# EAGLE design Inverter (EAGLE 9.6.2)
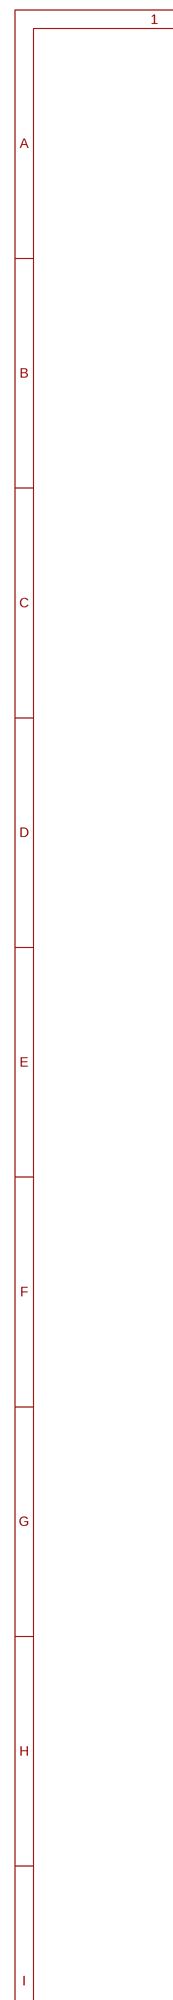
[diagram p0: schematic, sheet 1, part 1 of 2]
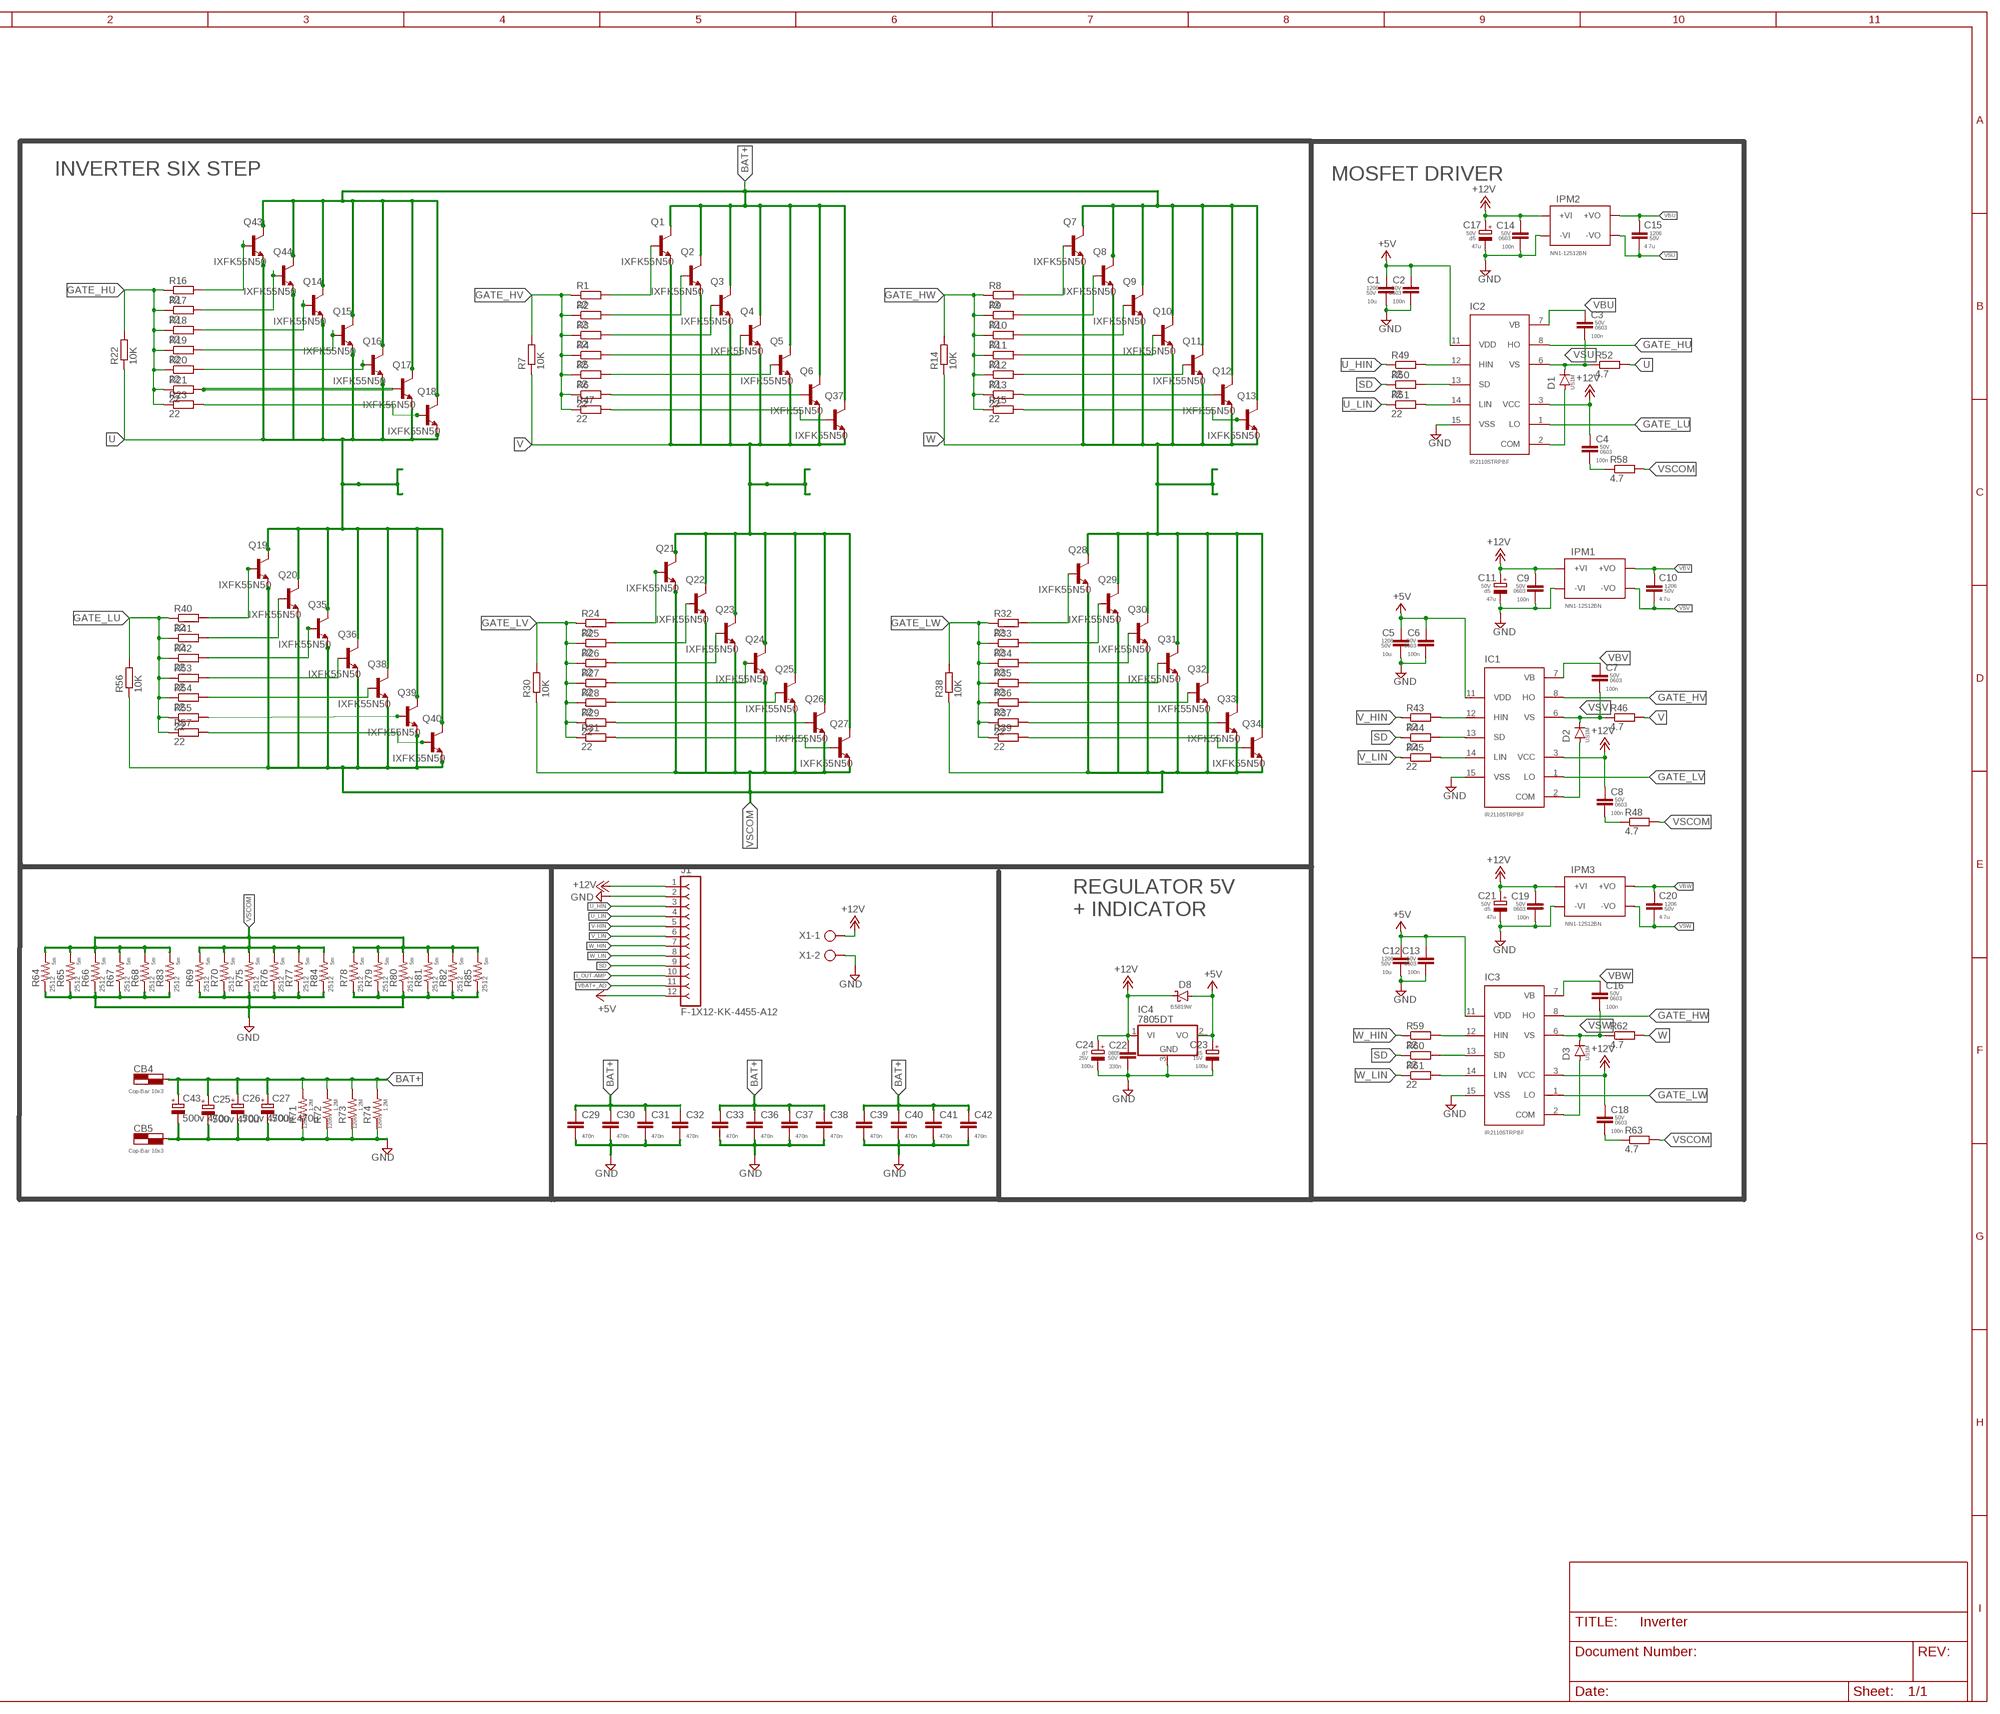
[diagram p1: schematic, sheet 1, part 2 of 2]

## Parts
C1  10u  C-EUC1206  [C1206]
C2  100n  C-EUC0603  [C0603]
C3  100n  C-EUC0603  [C0603]
C4  100n  C-EUC0603  [C0603]
C5  10u  C-EUC1206  [C1206]
C6  100n  C-EUC0603  [C0603]
C7  100n  C-EUC0603  [C0603]
C8  100n  C-EUC0603  [C0603]
C9  100n  C-EUC0603  [C0603]
C10  4.7u  C-EUC1206  [C1206]
C11  47u  CPOL-EUE2.5-5  [E2,5-5]
C12  10u  C-EUC1206  [C1206]
C13  100n  C-EUC0603  [C0603]
C14  100n  C-EUC0603  [C0603]
C15  4.7u  C-EUC1206  [C1206]
C16  100n  C-EUC0603  [C0603]
C17  47u  CPOL-EUE2.5-5  [E2,5-5]
C18  100n  C-EUC0603  [C0603]
C19  100n  C-EUC0603  [C0603]
C20  4.7u  C-EUC1206  [C1206]
C21  47u  CPOL-EUE2.5-5  [E2,5-5]
C22  330n  C-EUC0805  [C0805]
C23  100u  CPOL-EUE2.5-5  [E2,5-5]
C24  100u  CPOL-EUE2.5-7  [E2,5-7]
C25  500v 470u  CPOL-EUE10-35  [EB35D]
C26  500v 470u  CPOL-EUE10-35  [EB35D]
C27  500v 470u  CPOL-EUE10-35  [EB35D]
C29  470n  C-EU102-064X133  [C102-064X133]
C30  470n  C-EU102-064X133  [C102-064X133]
C31  470n  C-EU102-064X133  [C102-064X133]
C32  470n  C-EU102-064X133  [C102-064X133]
C33  470n  C-EU102-064X133  [C102-064X133]
C36  470n  C-EU102-064X133  [C102-064X133]
C37  470n  C-EU102-064X133  [C102-064X133]
C38  470n  C-EU102-064X133  [C102-064X133]
C39  470n  C-EU102-064X133  [C102-064X133]
C40  470n  C-EU102-064X133  [C102-064X133]
C41  470n  C-EU102-064X133  [C102-064X133]
C42  470n  C-EU102-064X133  [C102-064X133]
C43  500v 470u  CPOL-EUE10-35  [EB35D]
CB4  Cop-Bar 10x3  COOPPER_BAR15X2  [COP_BAR-15X2]
CB5  Cop-Bar 10x3  COOPPER_BAR15X2  [COP_BAR-15X2]
D1  US1M  GF1  [SMA-DO214AC]
D2  US1M  GF1  [SMA-DO214AC]
D3  US1M  GF1  [SMA-DO214AC]
D8  B5819W  SCHOTTKY-DIODESOD123  [DIODE_SOD123]
IC1  IR2110STRPBF  IR2110  [SO16W]
IC2  IR2110STRPBF  IR2110  [SO16W]
IC3  IR2110STRPBF  IR2110  [SO16W]
IC4  7805DT  [TO252]
IPM1  NN1-12S12BN  [NN1-12S12BN]
IPM2  NN1-12S12BN  [NN1-12S12BN]
IPM3  NN1-12S12BN  [NN1-12S12BN]
J1  F-1X12-KK-4455-A12  [KK-4455-A12]
Q1  IXFK55N50  2SC5200  [TO545P2020X520X2910-3]
Q2  IXFK55N50  2SC5200  [TO545P2020X520X2910-3]
Q3  IXFK55N50  2SC5200  [TO545P2020X520X2910-3]
Q4  IXFK55N50  2SC5200  [TO545P2020X520X2910-3]
Q5  IXFK55N50  2SC5200  [TO545P2020X520X2910-3]
Q6  IXFK55N50  2SC5200  [TO545P2020X520X2910-3]
Q7  IXFK55N50  2SC5200  [TO545P2020X520X2910-3]
Q8  IXFK55N50  2SC5200  [TO545P2020X520X2910-3]
Q9  IXFK55N50  2SC5200  [TO545P2020X520X2910-3]
Q10  IXFK55N50  2SC5200  [TO545P2020X520X2910-3]
Q11  IXFK55N50  2SC5200  [TO545P2020X520X2910-3]
Q12  IXFK55N50  2SC5200  [TO545P2020X520X2910-3]
Q13  IXFK55N50  2SC5200  [TO545P2020X520X2910-3]
Q14  IXFK55N50  2SC5200  [TO545P2020X520X2910-3]
Q15  IXFK55N50  2SC5200  [TO545P2020X520X2910-3]
Q16  IXFK55N50  2SC5200  [TO545P2020X520X2910-3]
Q17  IXFK55N50  2SC5200  [TO545P2020X520X2910-3]
Q18  IXFK55N50  2SC5200  [TO545P2020X520X2910-3]
Q19  IXFK55N50  2SC5200  [TO545P2020X520X2910-3]
Q20  IXFK55N50  2SC5200  [TO545P2020X520X2910-3]
Q21  IXFK55N50  2SC5200  [TO545P2020X520X2910-3]
Q22  IXFK55N50  2SC5200  [TO545P2020X520X2910-3]
Q23  IXFK55N50  2SC5200  [TO545P2020X520X2910-3]
Q24  IXFK55N50  2SC5200  [TO545P2020X520X2910-3]
Q25  IXFK55N50  2SC5200  [TO545P2020X520X2910-3]
Q26  IXFK55N50  2SC5200  [TO545P2020X520X2910-3]
Q27  IXFK55N50  2SC5200  [TO545P2020X520X2910-3]
Q28  IXFK55N50  2SC5200  [TO545P2020X520X2910-3]
Q29  IXFK55N50  2SC5200  [TO545P2020X520X2910-3]
Q30  IXFK55N50  2SC5200  [TO545P2020X520X2910-3]
Q31  IXFK55N50  2SC5200  [TO545P2020X520X2910-3]
Q32  IXFK55N50  2SC5200  [TO545P2020X520X2910-3]
Q33  IXFK55N50  2SC5200  [TO545P2020X520X2910-3]
Q34  IXFK55N50  2SC5200  [TO545P2020X520X2910-3]
Q35  IXFK55N50  2SC5200  [TO545P2020X520X2910-3]
Q36  IXFK55N50  2SC5200  [TO545P2020X520X2910-3]
Q37  IXFK55N50  2SC5200  [TO545P2020X520X2910-3]
Q38  IXFK55N50  2SC5200  [TO545P2020X520X2910-3]
Q39  IXFK55N50  2SC5200  [TO545P2020X520X2910-3]
Q40  IXFK55N50  2SC5200  [TO545P2020X520X2910-3]
Q43  IXFK55N50  2SC5200  [TO545P2020X520X2910-3]
Q44  IXFK55N50  2SC5200  [TO545P2020X520X2910-3]
R1  22  R-EU_R0805  [R0805]
R2  22  R-EU_R0805  [R0805]
R3  22  R-EU_R0805  [R0805]
R4  22  R-EU_R0805  [R0805]
R5  22  R-EU_R0805  [R0805]
R6  22  R-EU_R0805  [R0805]
R7  10K  R-EU_R0603  [R0603]
R8  22  R-EU_R0805  [R0805]
R9  22  R-EU_R0805  [R0805]
R10  22  R-EU_R0805  [R0805]
R11  22  R-EU_R0805  [R0805]
R12  22  R-EU_R0805  [R0805]
R13  22  R-EU_R0805  [R0805]
R14  10K  R-EU_R0603  [R0603]
R15  22  R-EU_R0805  [R0805]
R16  22  R-EU_R0805  [R0805]
R17  22  R-EU_R0805  [R0805]
R18  22  R-EU_R0805  [R0805]
R19  22  R-EU_R0805  [R0805]
R20  22  R-EU_R0805  [R0805]
R21  22  R-EU_R0805  [R0805]
R22  10K  R-EU_R0603  [R0603]
R23  22  R-EU_R0805  [R0805]
R24  22  R-EU_R0805  [R0805]
R25  22  R-EU_R0805  [R0805]
R26  22  R-EU_R0805  [R0805]
R27  22  R-EU_R0805  [R0805]
R28  22  R-EU_R0805  [R0805]
R29  22  R-EU_R0805  [R0805]
R30  10K  R-EU_R0603  [R0603]
R31  22  R-EU_R0805  [R0805]
R32  22  R-EU_R0805  [R0805]
R33  22  R-EU_R0805  [R0805]
R34  22  R-EU_R0805  [R0805]
R35  22  R-EU_R0805  [R0805]
R36  22  R-EU_R0805  [R0805]
R37  22  R-EU_R0805  [R0805]
R38  10K  R-EU_R0603  [R0603]
R39  22  R-EU_R0805  [R0805]
R40  22  R-EU_R0805  [R0805]
R41  22  R-EU_R0805  [R0805]
R42  22  R-EU_R0805  [R0805]
R43  22  R-EU_R0603  [R0603]
R44  22  R-EU_R0603  [R0603]
R45  22  R-EU_R0603  [R0603]
R46  4.7  R-EU_R0805  [R0805]
R47  22  R-EU_R0805  [R0805]
R48  4.7  R-EU_R0805  [R0805]
R49  22  R-EU_R0603  [R0603]
R50  22  R-EU_R0603  [R0603]
R51  22  R-EU_R0603  [R0603]
R52  4.7  R-EU_R0805  [R0805]
R53  22  R-EU_R0805  [R0805]
R54  22  R-EU_R0805  [R0805]
R55  22  R-EU_R0805  [R0805]
R56  10K  R-EU_R0603  [R0603]
R57  22  R-EU_R0805  [R0805]
R58  4.7  R-EU_R0805  [R0805]
R59  22  R-EU_R0603  [R0603]
R60  22  R-EU_R0603  [R0603]
R61  22  R-EU_R0603  [R0603]
R62  4.7  R-EU_R0805  [R0805]
R63  4.7  R-EU_R0805  [R0805]
R64  5m  R-US_R2512  [R2512]
R65  5m  R-US_R2512  [R2512]
R66  5m  R-US_R2512  [R2512]
R67  5m  R-US_R2512  [R2512]
R68  5m  R-US_R2512  [R2512]
R69  5m  R-US_R2512  [R2512]
R70  5m  R-US_R2512  [R2512]
R71  1.2M  R-US_R1206  [R1206]
R72  1.2M  R-US_R1206  [R1206]
R73  1.2M  R-US_R1206  [R1206]
R74  1.2M  R-US_R1206  [R1206]
R75  5m  R-US_R2512  [R2512]
R76  5m  R-US_R2512  [R2512]
R77  5m  R-US_R2512  [R2512]
R78  5m  R-US_R2512  [R2512]
R79  5m  R-US_R2512  [R2512]
R80  5m  R-US_R2512  [R2512]
R81  5m  R-US_R2512  [R2512]
R82  5m  R-US_R2512  [R2512]
R83  5m  R-US_R2512  [R2512]
R84  5m  R-US_R2512  [R2512]
R85  5m  R-US_R2512  [R2512]
X1  AK500/2  [AK500/2]

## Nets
+5V: C1.1 C2.1 C5.1 C6.1 C12.1 C13.1 C23.+ D8.A IC1.11(VDD) IC2.11(VDD) IC3.11(VDD) IC4.2(VO) J1.12
+12V: C9.1 C11.+ C14.1 C17.+ C19.1 C21.+ C22.1 C24.+ D8.C IC4.1(VI) IPM1.1(+VI) IPM2.1(+VI) IPM3.1(+VI) J1.1 X1.1
BAT+: C25.+ C26.+ C27.+ C29.1 C30.1 C31.1 C32.1 C33.1 C36.1 C37.1 C38.1 C39.1 C40.1 C41.1 C42.1 C43.+ CB4.P$1 Q1.2(C) Q2.2(C) Q3.2(C) Q4.2(C) Q5.2(C) Q6.2(C) Q7.2(C) Q8.2(C) Q9.2(C) Q10.2(C) Q11.2(C) Q12.2(C) Q13.2(C) Q14.2(C) Q15.2(C) Q16.2(C) Q17.2(C) Q18.2(C) Q37.2(C) Q43.2(C) Q44.2(C) R71.2 R72.2 R73.2 R74.2
COM: D1.A D2.A D3.A IC1.2(COM) IC2.2(COM) IC3.2(COM)
GATE_HU: IC2.8(HO) R16.1 R17.1 R18.1 R19.1 R20.1 R21.1 R22.2 R23.1
GATE_HV: IC1.8(HO) R1.1 R2.1 R3.1 R4.1 R5.1 R6.1 R7.2 R47.1
GATE_HW: IC3.8(HO) R8.1 R9.1 R10.1 R11.1 R12.1 R13.1 R14.2 R15.1
GATE_LU: IC2.1(LO) R40.1 R41.1 R42.1 R53.1 R54.1 R55.1 R56.2 R57.1
GATE_LV: IC1.1(LO) R24.1 R25.1 R26.1 R27.1 R28.1 R29.1 R30.2 R31.1
GATE_LW: IC3.1(LO) R32.1 R33.1 R34.1 R35.1 R36.1 R37.1 R38.2 R39.1
GND: C1.2 C2.2 C5.2 C6.2 C9.2 C11.- C12.2 C13.2 C14.2 C17.- C19.2 C21.- C22.2 C23.- C24.- C25.- C26.- C27.- C29.2 C30.2 C31.2 C32.2 C33.2 C36.2 C37.2 C38.2 C39.2 C40.2 C41.2 C42.2 C43.- CB5.P$1 IC1.15(VSS) IC2.15(VSS) IC3.15(VSS) IC4.3(GND) IPM1.2(-VI) IPM2.2(-VI) IPM3.2(-VI) J1.2 R64.1 R65.1 R66.1 R67.1 R68.1 R69.1 R70.1 R71.1 R72.1 R73.1 R74.1 R75.1 R76.1 R77.1 R78.1 R79.1 R80.1 R81.1 R82.1 R83.1 R84.1 R85.1 X1.2
I_OUT-AMP: J1.10
N$1: IC1.12(HIN) R43.2
N$2: IC1.13(SD) R44.2
N$3: Q1.1(B) R1.2
N$4: Q2.1(B) R2.2
N$5: Q3.1(B) R3.2
N$6: Q4.1(B) R4.2
N$7: Q5.1(B) R5.2
N$8: Q6.1(B) R6.2
N$9: IC3.12(HIN) R59.2
N$10: Q7.1(B) R8.2
N$11: Q8.1(B) R9.2
N$12: Q9.1(B) R10.2
N$13: Q10.1(B) R11.2
N$14: Q11.1(B) R12.2
N$15: Q12.1(B) R13.2
N$17: Q13.1(B) R15.2
N$19: IC1.14(LIN) R45.2
N$20: Q43.1(B) R16.2
N$21: Q44.1(B) R17.2
N$22: Q14.1(B) R18.2
N$23: Q15.1(B) R19.2
N$24: Q16.1(B) R20.2
N$25: Q17.1(B) R21.2
N$26: C8.2 R48.1
N$27: Q18.1(B) R23.2
N$28: IC3.13(SD) R60.2
N$29: IC3.14(LIN) R61.2
N$30: Q21.1(B) R24.2
N$31: Q22.1(B) R25.2
N$32: Q23.1(B) R26.2
N$33: Q24.1(B) R27.2
N$34: Q25.1(B) R28.2
N$35: Q26.1(B) R29.2
N$36: C18.2 R63.1
N$37: Q27.1(B) R31.2
N$40: Q28.1(B) R32.2
N$41: Q29.1(B) R33.2
N$42: Q30.1(B) R34.2
N$43: Q31.1(B) R35.2
N$44: Q32.1(B) R36.2
N$45: Q33.1(B) R37.2
N$47: Q34.1(B) R39.2
N$50: Q19.1(B) R40.2
N$51: Q20.1(B) R41.2
N$52: Q35.1(B) R42.2
N$53: Q36.1(B) R53.2
N$54: Q38.1(B) R54.2
N$58: Q37.1(B) R47.2
N$59: IC2.12(HIN) R49.2
N$60: IC2.13(SD) R50.2
N$61: IC2.14(LIN) R51.2
N$63: Q39.1(B) R55.2
N$65: Q40.1(B) R57.2
N$67: C4.2 R58.1
SD: J1.9 R44.1 R50.1 R60.1
U: Q14.3(E) Q15.3(E) Q16.3(E) Q18.3(E) Q19.2(C) Q20.2(C) Q35.2(C) Q36.2(C) Q38.2(C) Q39.2(C) Q40.2(C) Q43.3(E) Q44.3(E) R22.1 R52.2
U_HIN: J1.3 R49.1
U_LIN: J1.4 R51.1
V: Q1.3(E) Q2.3(E) Q3.3(E) Q4.3(E) Q5.3(E) Q6.3(E) Q21.2(C) Q22.2(C) Q23.2(C) Q24.2(C) Q25.2(C) Q26.2(C) Q27.2(C) Q37.3(E) R7.1 R46.2
V-HIN: J1.5
V_HIN: R43.1
V_LIN: J1.6 R45.1
VBAT+_AD: J1.11
VBU: C3.1 C15.1 IC2.7(VB) IPM2.6(+VO)
VBV: C7.1 C10.1 IC1.7(VB) IPM1.6(+VO)
VBW: C16.1 C20.1 IC3.7(VB) IPM3.6(+VO)
VCC: C4.1 C8.1 C18.1 IC1.3(VCC) IC2.3(VCC) IC3.3(VCC) ; supply symbol labelled +12V
VSCOM: Q19.3(E) Q20.3(E) Q21.3(E) Q22.3(E) Q23.3(E) Q24.3(E) Q25.3(E) Q26.3(E) Q27.3(E) Q28.3(E) Q29.3(E) Q30.3(E) Q31.3(E) Q32.3(E) Q33.3(E) Q34.3(E) Q35.3(E) Q36.3(E) Q38.3(E) Q39.3(E) Q40.3(E) R30.1 R38.1 R48.2 R56.1 R58.2 R63.2 R64.2 R65.2 R66.2 R67.2 R68.2 R69.2 R70.2 R75.2 R76.2 R77.2 R78.2 R79.2 R80.2 R81.2 R82.2 R83.2 R84.2 R85.2
VSU: C3.2 C15.2 D1.K(C) IC2.6(VS) IPM2.4(-VO) R52.1
VSV: C7.2 C10.2 D2.K(C) IC1.6(VS) IPM1.4(-VO) R46.1
VSW: C16.2 C20.2 D3.K(C) IC3.6(VS) IPM3.4(-VO) R62.1
W: Q7.3(E) Q8.3(E) Q9.3(E) Q10.3(E) Q11.3(E) Q12.3(E) Q13.3(E) Q28.2(C) Q29.2(C) Q30.2(C) Q31.2(C) Q32.2(C) Q33.2(C) Q34.2(C) R14.1 R62.2
W_HIN: J1.7 R59.1
W_LIN: J1.8 R61.1
Unconnected: Q17.3(E)

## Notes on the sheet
- INVERTER SIX STEP | MOSFET DRIVER
- REGULATOR 5V 
  + INDICATOR

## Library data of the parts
C1 C5 C10 C12 C15 C20 = rcl:C-EU: CAPACITOR, European symbol; SIZE: 1206; SPICEPREFIX: C; VOLTAGE: 50V
C2-C4 C6-C9 C13 C14 C16 C18 C19 = rcl:C-EU: CAPACITOR, European symbol; SIZE: 0603; SPICEPREFIX: C; VOLTAGE: 50V
C11 C17 C21 = rcl:CPOL-EU: POLARIZED CAPACITOR, European symbol; DIAMETER: d5; SPICEPREFIX: C; VOLTAGE: 50V
C22 = rcl:C-EU: CAPACITOR, European symbol; SIZE: 0805; SPICEPREFIX: C; VOLTAGE: 50V
C23 = rcl:CPOL-EU: POLARIZED CAPACITOR, European symbol; DIAMETER: d5; SPICEPREFIX: C; VOLTAGE: 15V
C24 = rcl:CPOL-EU: POLARIZED CAPACITOR, European symbol; SIZE: d7; SPICEPREFIX: C; VOLTAGE: 25V
C25-C27 C43 = rcl:CPOL-EU: POLARIZED CAPACITOR, European symbol; SPICEPREFIX: C
C29-C33 C36-C42 = rcl:C-EU: CAPACITOR, European symbol; SPICEPREFIX: C
CB4 CB5 = power-connector:COOPPER_BAR
D1-D3 = diode:GF1: DIODE
D8 = diode:SCHOTTKY-DIODE: Schottky Diode
IC1-IC3 = irs:IR2110
IC4 = linear:78*: Positive VOLTAGE REGULATOR Source: http://cache.national.com/ds/LM/LM78L05.pdf http://www.fairchildsemi.com/ds/LM/LM7805.pdf
IPM1-IPM3 = Isolated-Power-Module:NN1-12S12BN: 12V to 12V 200mW isolated Power Module
J1 = con-headers-jp:F-1X12-: FEMALE HEADER
Q1-Q40 Q43 Q44 = 2SC5200:2SC5200: 2SC5200 Series NPN 230 V 15 A Epitaxial Planar Bipolar Transistor - TO-264 Check availability; AVAILABILITY: In Stock; DESCRIPTION: Bipolar (BJT) Transistor NPN 230 V 15 A 30MHz 150 W Through Hole TO-264; MF: STMicroelectronics; MP: 2SC5200; PACKAGE: TO-264-3 STMicroelectronics; PRICE: None; PURCHASE-URL: https://pricing.snapeda.com/search/part/2SC5200/?ref=eda
R1-R63 = rcl:R-EU_: RESISTOR, European symbol; SPICEPREFIX: R
R64-R70 R75-R85 = rcl:R-US_: RESISTOR, American symbol; SIZE: 2512; SPICEPREFIX: R
R71-R74 = rcl:R-US_: RESISTOR, American symbol; SIZE: 1206; SPICEPREFIX: R
X1 = con-ptr500:AK500/2: CONNECTOR; OC_FARNELL: unknown; OC_NEWARK: unknown

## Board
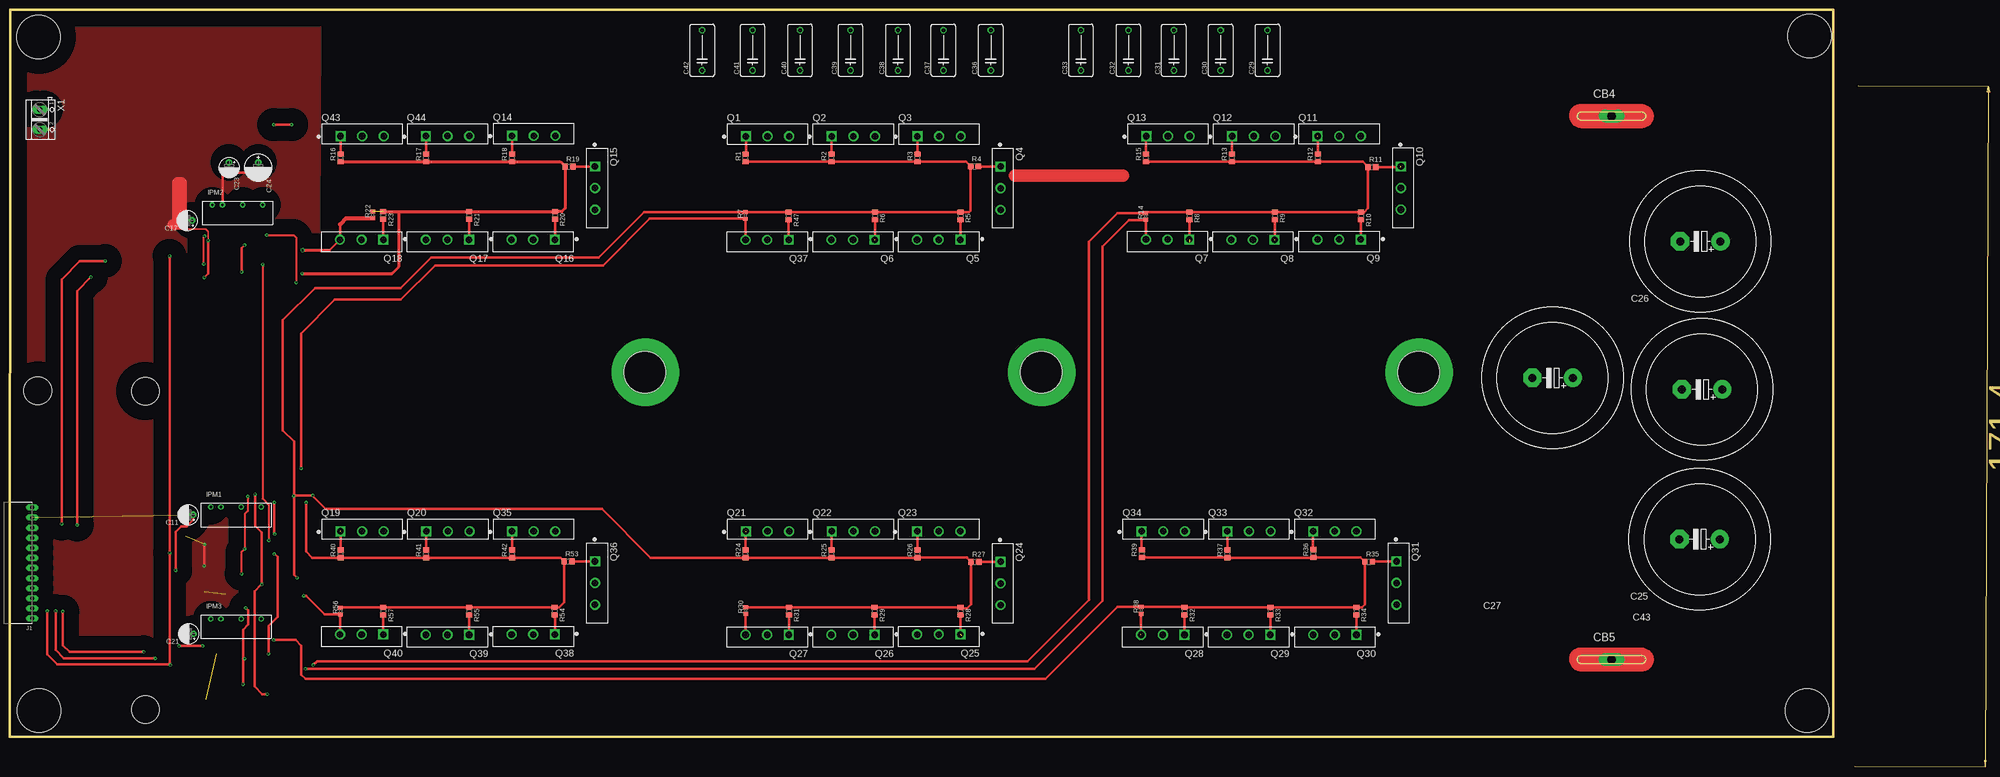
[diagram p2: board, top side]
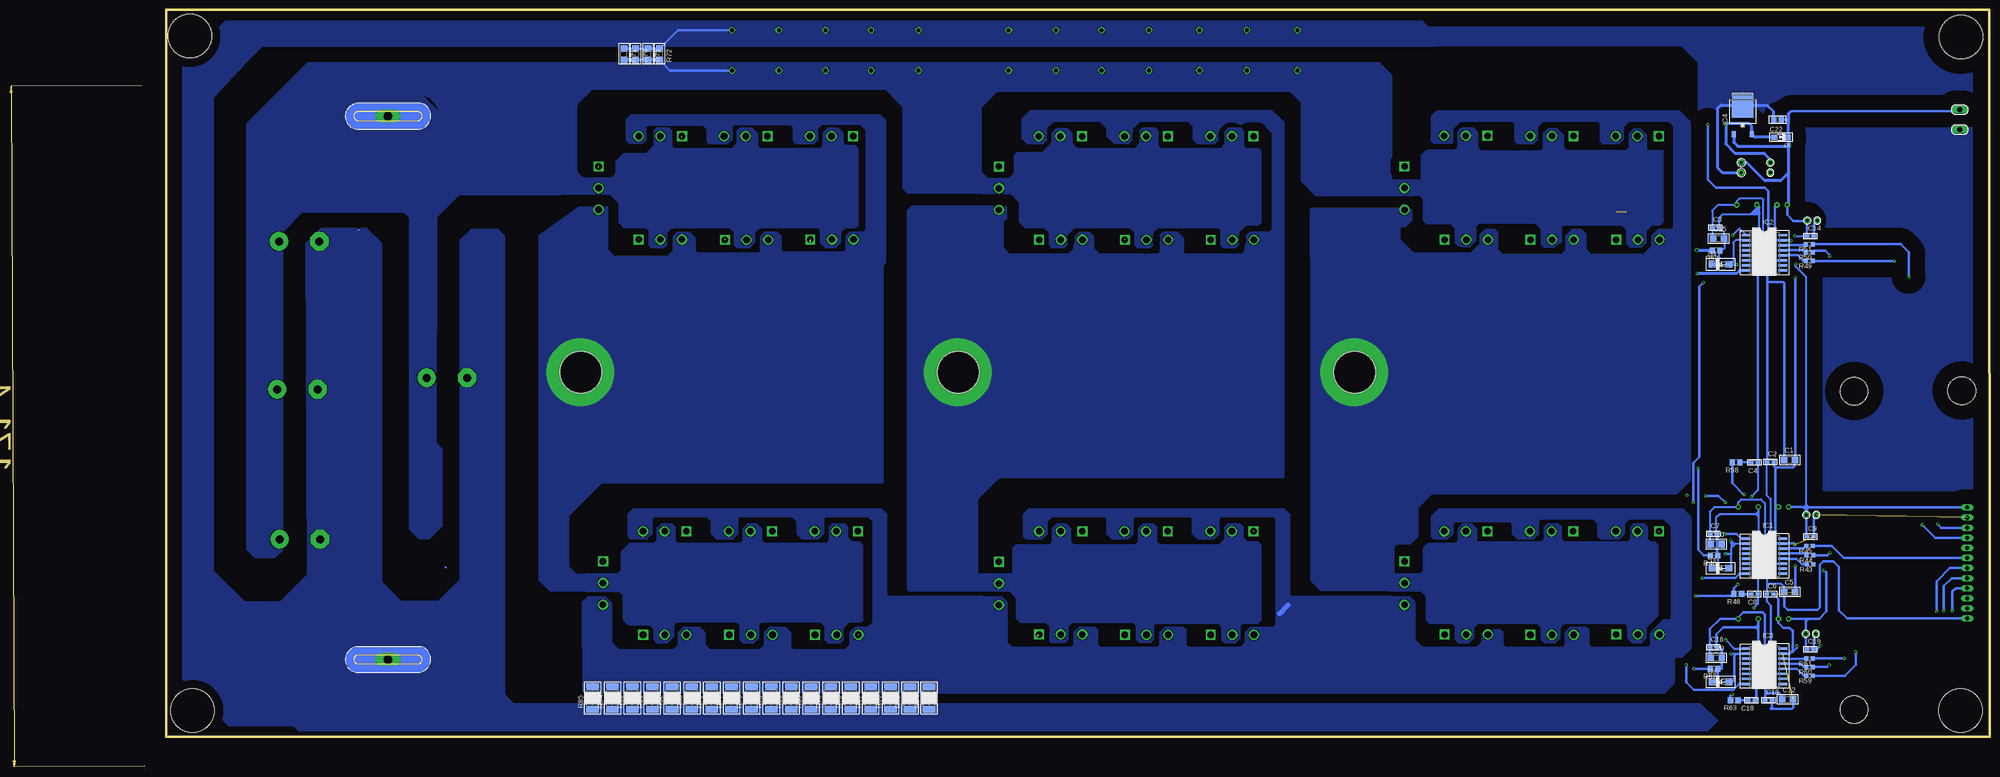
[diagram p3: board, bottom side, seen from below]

Size 498.4 x 190.65 mm. Coordinates in mm from the lower left corner, seen from the top.
Outline: 0,7.55 459.1,7.55 459.1,190.65 0.1,190.65 0,7.55
Outline: 0,7.55 0,7.65
Copper layers (1*16): Top 0.035mm / dielectric 1.5mm / Bottom 0.035mm
Design rules "default": minimum track width 6mil, minimum drill 0.35mm, track to track 6mil, track to pad 6mil, pad to pad 6mil, via to via 6mil, smd to smd 6mil, copper to edge 40mil, drill to drill 6mil, minimum pad ring 10mil, minimum via ring 8mil, stop-mask expansion 4mil, vias tented up to drill 0mil, thermal gap 10mil
Holes 10.5 mm at 159.81,99.38 259.67,99.38 354.67,99.38
Holes 7 mm at 34.1,14.45 34.1,94.65 7,94.75
Holes 11 mm at 7.3,14.15 7.2,183.85 453.1,184.05 452.4,14.15

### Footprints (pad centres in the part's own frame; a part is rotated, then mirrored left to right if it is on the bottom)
C1206 = smd 1.6 x 1.8: 1 -1.4,0; 2 1.4,0
C0603 = smd 1.1 x 1: 1 -0.85,0; 2 0.85,0
E2,5-5 = drill 0.813 pad 1.6: + -1.27,0 | drill 0.813 pad 1.6 octagon: - 1.27,0
C0805 = smd 1.3 x 1.5: 1 -0.95,0; 2 0.95,0
E2,5-7 = drill 0.813 pad 1.6: + -1.27,0 | drill 0.813 pad 1.6 octagon: - 1.27,0
EB35D = drill 2.007 pad 4.597: + -5.08,0 | drill 2.007 pad 4.597 octagon: - 5.08,0
C102-064X133 = drill 1.016 octagon: 1 -5.08,0; 2 5.08,0
COP_BAR-15X2 = drill 2.2 long: P$1 0,0
SMA-DO214AC = smd 1.8 x 1.7: A 2.05,0; K -2.05,0
DIODE_SOD123 = smd 1.4 x 1.4: A 1.805,0; C -1.805,0
SO16W = smd 0.6 x 2.2: 1 -4.445,-4.6; 2 -3.175,-4.6; 3 -1.905,-4.6; 4 -0.635,-4.6; 5 0.635,-4.6; 6 1.905,-4.6; 7 3.175,-4.6; 8 4.445,-4.6; 9 4.445,4.6; 10 3.175,4.6; 11 1.905,4.6; 12 0.635,4.6; 13 -0.635,4.6; 14 -1.905,4.6; 15 -3.175,4.6; 16 -4.445,4.6
TO252 = smd 1 x 1.6: 1 -2.28,-4.8; 2 2.28,-4.8 | smd 5.4 x 6.2: 3 0,2.5
NN1-12S12BN = drill 0.7 pad 1.27: 1 -6.35,2.54; 2 -3.81,2.54; 4 1.27,2.54; 6 6.35,2.54
KK-4455-A12 = drill 1.067 long: 1 -13.97,0; 2 -11.43,0; 3 -8.89,0; 4 -6.35,0; 5 -3.81,0; 6 -1.27,0; 7 1.27,0; 8 3.81,0; 9 6.35,0; 10 8.89,0; 11 11.43,0; 12 13.97,0
TO545P2020X520X2910-3 = drill 1.66 square: 1 0,0 | drill 1.66: 2 5.45,0; 3 10.9,0
R0805 = smd 1.3 x 1.5: 1 -0.95,0; 2 0.95,0
R0603 = smd 1 x 1.1: 1 -0.85,0; 2 0.85,0
R2512 = smd 1.8 x 3.2: 1 -2.8,0; 2 2.8,0
R1206 = smd 1.6 x 1.803: 1 -1.422,0; 2 1.422,0
AK500/2 = drill 1.321 long: 1 -2.515,0; 2 2.515,0

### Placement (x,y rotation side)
C1  50.33,77.34 0 bottom
C2  55.16,76.83 0 bottom
C3  69,135.84 0 bottom
C4  59.16,76.65 180 bottom
C5  50.33,44.12 0 bottom
C6  55.23,43.52 0 bottom
C7  69.59,58.69 0 bottom
C8  59.2,43.52 180 bottom
C9  45.12,57.99 0 bottom
C10  68.8,56.11 0 bottom
C11  44.87,63.5 180 top
C12  50.86,17 0 bottom
C13  55.64,16.8 0 bottom
C14  45.12,133.68 0 bottom
C15  68.24,133.04 0 bottom
C16  69.59,30.1 0 bottom
C17  44.62,137.61 180 top
C18  59.96,16.8 180 bottom
C19  45.12,29.6 0 bottom
C20  68.8,27.5 0 bottom
C21  45.01,33.52 180 top
C22  53.38,163.01 180 bottom
C23  55.16,150.95 270 top
C24  62.52,150.95 270 top
C25  425.41,57.35 180 top
C26  425.58,132.35 180 top
C27  388.38,97.98 180 top
C29  316.63,180.49 90 top
C30  304.82,180.49 90 top
C31  293.01,180.49 90 top
C32  281.58,180.49 90 top
C33  269.64,180.49 90 top
C36  246.94,180.49 90 top
C37  235,180.49 90 top
C38  223.57,180.49 90 top
C39  211.63,180.49 90 top
C40  198.93,180.49 90 top
C41  187,180.49 90 top
C42  174.3,180.49 90 top
C43  426.01,95.08 180 top
CB4  403.23,163.9 0 top
CB5  403.23,27.05 0 top
D1  67.73,126.57 0 bottom
D2  67.73,50.04 0 bottom
D3  67.73,21.4 0 bottom
D8  52.49,158.57 180 bottom
IC1  56.68,53.09 270 bottom
IC2  56.68,129.49 270 bottom
IC3  56.68,25.35 270 bottom
IC4  62.14,164.16 0 bottom
IPM1  56.94,62.95 0 top
IPM2  57.32,139.01 0 top
IPM3  56.94,34.78 0 top
J1  5.6,51.35 270 top
Q1  185.3,158.82 0 top
Q2  206.89,158.82 0 top
Q3  228.48,158.82 0 top
Q4  249.44,151.2 270 top
Q5  239.28,132.79 180 top
Q6  217.7,132.75 180 top
Q7  296.9,132.85 180 top
Q8  318.4,132.75 180 top
Q9  340.1,132.85 180 top
Q10  350.2,151.25 270 top
Q11  329.2,158.85 0 top
Q12  307.7,158.85 0 top
Q13  286.1,158.85 0 top
Q14  126.42,158.95 0 top
Q15  147.29,151.23 270 top
Q16  137.18,132.77 180 top
Q17  115.58,132.78 180 top
Q18  93.98,132.79 180 top
Q19  83.2,59.35 0 top
Q20  104.8,59.35 0 top
Q21  185.3,59.35 0 top
Q22  206.9,59.35 0 top
Q23  228.4,59.35 0 top
Q24  249.4,51.65 270 top
Q25  239.3,33.35 180 top
Q26  217.7,33.25 180 top
Q27  196.1,33.25 180 top
Q28  295.7,33.25 180 top
Q29  317.3,33.25 180 top
Q30  339,33.25 180 top
Q31  349.1,51.75 270 top
Q32  328.1,59.35 0 top
Q33  306.5,59.35 0 top
Q34  284.9,59.35 0 top
Q35  126.4,59.35 0 top
Q36  147.3,51.75 270 top
Q37  196.1,132.75 180 top
Q38  137.2,33.35 180 top
Q39  115.6,33.25 180 top
Q40  94,33.35 180 top
Q43  83.23,158.85 0 top
Q44  104.73,158.87 0 top
R1  185.25,153.36 90 top
R2  206.83,153.4 90 top
R3  228.51,153.4 90 top
R4  242.84,151.24 0 top
R5  239.31,138.75 270 top
R6  217.76,138.75 270 top
R7  185.14,138.88 90 top
R8  296.95,138.75 270 top
R9  318.45,138.75 270 top
R10  340.15,138.75 270 top
R11  342.89,151.1 0 top
R12  329.25,153.4 90 top
R13  307.65,153.4 90 top
R14  285.95,138.65 90 top
R15  286.05,153.4 90 top
R16  83.22,153.36 90 top
R17  104.81,153.36 90 top
R18  126.4,153.36 90 top
R19  140.76,151.2 0 top
R20  137.2,138.88 270 top
R21  115.61,138.88 270 top
R22  91.35,139.01 90 top
R23  94.02,138.88 270 top
R24  185.26,53.65 90 top
R25  206.85,53.65 90 top
R26  228.49,53.65 90 top
R27  242.95,51.63 0 top
R28  239.36,39.25 270 top
R29  217.71,39.25 270 top
R30  185.26,39.35 90 top
R31  196.11,39.25 270 top
R32  295.75,39.25 270 top
R33  317.35,39.25 270 top
R34  338.95,39.25 270 top
R35  342.09,51.7 0 top
R36  328.15,53.75 90 top
R37  306.55,53.65 90 top
R38  284.8,39.45 90 top
R39  284.95,53.69 90 top
R40  83.25,53.65 90 top
R41  104.77,53.65 90 top
R42  126.4,53.65 90 top
R43  45.18,51.01 180 bottom
R44  45.25,53.3 180 bottom
R45  45.35,55.68 180 bottom
R46  69.38,53.21 180 bottom
R47  196.08,138.75 270 top
R48  63.4,43.53 180 bottom
R49  45.38,127.45 180 bottom
R50  45.38,129.61 180 bottom
R51  45.38,131.65 180 bottom
R52  68.87,129.99 180 bottom
R53  140.51,51.75 0 top
R54  137.14,39.25 270 top
R55  115.61,39.25 270 top
R56  83.24,39.25 90 top
R57  94.02,39.25 270 top
R58  63.79,76.66 180 bottom
R59  45.35,22.95 180 bottom
R60  45.35,25.15 180 bottom
R61  45.35,27.27 180 bottom
R62  69.38,24.72 180 bottom
R63  64.26,16.82 180 bottom
R64  267,17.35 90 bottom
R65  271.8,17.35 90 bottom
R66  276.7,17.35 90 bottom
R67  281.7,17.35 90 bottom
R68  301.7,17.35 90 bottom
R69  296.7,17.35 90 bottom
R70  291.7,17.35 90 bottom
R71  343.82,179.51 270 bottom
R72  334.87,179.51 270 bottom
R73  337.77,179.51 270 bottom
R74  340.87,179.51 270 bottom
R75  286.7,17.35 90 bottom
R76  321.7,17.35 90 bottom
R77  316.7,17.35 90 bottom
R78  311.7,17.35 90 bottom
R79  306.7,17.35 90 bottom
R80  341.7,17.35 90 bottom
R81  336.7,17.35 90 bottom
R82  331.7,17.35 90 bottom
R83  326.7,17.35 90 bottom
R84  346.7,17.35 90 bottom
R85  351.7,17.35 90 bottom
X1  7.53,163.02 270 top

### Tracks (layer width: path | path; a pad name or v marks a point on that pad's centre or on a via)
+5V  (via drill 0.35)
  Top 0.61: v70.91,161.74 v66.46,161.74
  Bottom 0.508: IC1.11 52.11,51.15 54.55,51.15 | 54.55,51.15 55.05,51.15 | 55.05,51.15 55.3,51.15 56.08,50.37 56.08,45.65 | 56.08,45.65 C6.1 | 55.05,51.15 55.05,51.65 | 55.05,51.65 55.05,67.4 56.05,68.4 56.05,76.79 C2.1 | 55.05,51.65 54.55,51.15 | C5.1 51.73,45.34 52.55,46.15 55.58,46.15 56.08,45.65
  Bottom 0.61: C2.1 56.01,122.15 | 56.01,122.15 56.01,126.6 55.67,126.95 | 55.67,126.95 55.03,127.58 IC2.11 | 55.67,126.95 55.67,144.98 56.55,145.87 68.87,145.87 70.91,147.9 v70.91,161.74 | C1.1 51.73,121.84 52.05,122.15 56.01,122.15 | C13.1 56.49,18.05 | 56.49,18.05 56.49,18.55 | 56.49,18.55 56.49,19.25 | 56.49,19.25 56.49,21.76 55.05,23.2 | IC3.11 54.8,23.45 55.05,23.2 | C12.1 52.26,17.91 53,18.65 55.89,18.65 | 55.89,18.65 56.39,18.65 56.49,18.55 | 56.49,19.25 55.89,18.65 | 55.89,18.65 56.49,18.05 | C6.1 56.08,41.63 55.05,40.6 55.05,23.2 | J1.12 35.83,37.38 37.9,39.45 37.9,50.35 39.3,51.75 41.9,51.75 42.8,50.85 42.8,40.15 43.4,39.55 50.8,39.55 51.73,40.49 C5.1
  Bottom 0.813: D8.A 59.08,158.57 IC4.2 59.86,161.37 60.49,162 66.21,162 v66.46,161.74 66.46,156.92 64.17,154.63 56.81,154.63 55.16,152.98 C23.+
+12V  (via drill 0.35)
  Top 0.508: v48.81,126.7 48.81,133.44 v49.01,133.64
  Top 0.61: v41.7,49.55 41.7,59.15 43.1,60.55 44.5,60.55 46.14,62.19 C11.+
  Bottom 0.508: C11.+ 46.14,65.05 46.14,65.95 | 46.14,65.95 46.14,123.36 48.87,126.09 48.87,126.64 v48.81,126.7 | v49.01,133.64 48.98,133.68 C14.1 | 46.14,65.95 46.62,65.47 46.62,65.23 | 46.14,65.95 45.6,65.41 45.6,65.32
  Bottom 0.61: 46.01,133.72 C14.1 45.97,137.53 | C17.+ 45.97,137.53 | IPM2.1 50.97,139.14 49.36,137.53 45.97,137.53 | 46.3,64.9 46.3,63.66 C11.+ 46.14,58.16 C9.1 | 46.88,65.49 46.62,65.23 46.3,64.9 | IPM1.1 46.88,65.49 | IPM3.1 46.4,37.32 | 46.4,37.32 45.56,37.32 | 45.56,37.32 42.93,37.32 41.1,39.15 41.1,48.95 v41.7,49.55 | C19.1 46.28,29.91 C21.+ 46.28,37.2 | 46.28,37.2 45.98,36.9 45.56,37.32 | 46.28,37.2 46.4,37.32 | 50.33,164.79 49.91,165.21 7.85,165.21 X1.1 | J1.1 45.6,65.32 | 45.6,65.32 45.87,65.32 46.14,65.05 | 46.88,65.49 45.76,65.49 45.6,65.32 | 46.3,64.9 46.02,64.9 45.6,65.32
  Bottom 0.813: IC4.1 64.42,157.29 63.41,156.28 50.97,156.28 50.69,156.56 | 50.69,156.56 D8.C 50.69,162.25 | 50.69,162.25 50.69,162.61 51.09,163.01 C22.1 | 50.33,164.79 50.71,164.41 50.71,162.28 50.69,162.25 | 62.4,152.35 C24.+ 61.13,152.22 56.55,147.65 52.62,147.65 50.69,149.58 | 50.69,156.56 50.69,149.58 | 50.69,149.58 50.69,141.83 IPM2.1
BAT+
  Bottom 0.61: R71.2 R74.2 R73.2 R72.2 332.19,175.41 C29.1
  pour Bottom: 86.65,132.03 87.8,130.88 90.34,130.88 91.23,131.77 91.23,135.2 92.5,136.47 107.59,136.47 107.99,136.07 107.99,132.15 109.77,130.88 112.05,130.88 112.69,131.52 112.69,135.46 114.21,136.98 128.56,136.98 129.58,135.96 129.58,132.41 130.98,131.01 132.88,131.01 133.14,131.26 133.64,131.26 134.41,132.03 134.41,135.58 135.68,136.85 141.65,136.85 142.41,137.61 142.41,142.99 143.49,144.06 152.69,144.06 152.69,147.01 151.93,147.77 142.92,147.77 142.92,154.12 141.65,155.39 134.53,155.39 133.79,156.14 133.79,159.91 132.85,160.86 129.96,160.86 129.07,159.97 129.07,156.16 128.06,155.14 112.94,155.14 112.25,155.83 112.25,159.56 111.08,160.73 109.01,160.73 107.48,159.2 107.48,155.9 106.85,155.27 91.23,155.27 90.54,155.96 90.54,159.63 89.57,160.6 87.92,160.6 86.53,159.2 86.53,155.78 86.02,155.27 82.34,155.27 82.34,137.23 83.1,136.47 85.13,136.47 86.65,134.95
  pour Bottom: 354.69,148.16 354.69,144.47 354.55,144.34 347.25,144.34 345.1,142.18 345.1,137.17 343.89,135.96 338.18,135.96 337.54,135.33 337.54,131.52 336.91,130.88 333.73,130.88 333.1,131.52 333.1,134.69 331.82,135.96 317.22,135.96 315.95,134.69 315.95,131.52 315.31,130.88 312.14,130.88 310.87,132.15 310.87,134.69 309.6,135.96 295,135.96 294.36,135.33 294.36,132.15 293.09,130.88 290.55,130.88 289.28,132.15 289.28,134.69 288.01,135.96 285.47,135.96 284.84,136.6 284.84,155.65 285.47,156.28 288.01,156.28 288.65,156.92 288.65,159.46 289.92,160.73 292.45,160.73 293.73,159.46 293.73,156.28 294.36,155.65 309.6,155.65 310.24,156.28 310.24,159.46 311.5,160.73 314.68,160.73 315.31,160.09 315.31,156.92 316.59,155.65 331.19,155.65 331.82,156.28 331.82,160.09 332.46,160.73 335.63,160.73 336.27,160.09 336.27,156.28 338.18,154.38 343.89,154.38 345.8,152.47 345.8,149.3 346.94,148.16
  pour Bottom: 253.88,147.39 253.88,144.85 253.49,144.46 246.4,144.46 244.23,142.29 244.23,137.33 242.86,135.96 238.01,135.96 236.74,134.69 236.74,131.52 236.1,130.88 232.93,130.88 232.29,131.52 232.29,134.06 230.39,135.96 216.42,135.96 215.15,134.69 215.15,131.52 214.51,130.88 211.34,130.88 210.7,131.52 210.7,134.69 209.43,135.96 194.19,135.96 193.56,135.33 193.56,131.52 192.92,130.88 189.75,130.88 189.11,131.52 189.11,134.69 187.21,136.6 184.03,136.6 183.4,137.23 183.4,155.01 184.03,155.65 187.21,155.65 187.84,156.28 187.84,160.09 188.48,160.73 191.65,160.73 192.54,159.84 192.54,156.66 193.56,155.65 208.8,155.65 209.43,156.28 209.43,160.09 210.06,160.73 213.24,160.73 213.88,160.09 213.88,156.92 215.15,155.65 229.75,155.65 231.02,156.92 231.02,159.46 232.16,160.6 234.96,160.6 236.1,159.46 236.1,156.92 238.39,154.63 244.86,154.63 245.5,154 245.5,149.43 246.9,148.03 253.25,148.03
  pour Bottom (isolate 2.184): 150.54,147.52 150.54,174.19 153.58,177.24 423.42,177.24 438.81,161.85 438.81,144.39 350.24,144.39 346.94,147.69 346.94,147.9 353.8,147.9 355.7,149.81 355.7,166.95 351.84,170.81 278.01,170.81 273.53,166.33 273.53,145.74 272.45,144.66 247.02,144.66 247.02,147.52 247.78,148.28 252.36,148.28 253.88,149.81 253.88,166.19 249.79,170.28 176.16,170.28 173.31,167.43 173.31,147.7 169.67,144.06 144.85,144.06 144.44,144.47 144.44,146.76 145.2,147.52
  pour Bottom: 438.82,143.91 438.82,54.9 436.77,52.85 431.62,52.85 429.79,54.68 429.79,134.88 424.77,139.9 399.26,139.9 397.81,138.44 397.81,84.96 397.75,59.93 395.48,57.66 392.7,57.66 389.57,60.79 389.57,80 391.07,81.49 391,138.59 385.29,144.3 359.78,144.3 357.86,145.76 371.13,145.55 398.37,172.79 409.93,172.79
COM  (via drill 0.35)
  Top 0.508: v63.63,126.53 63.63,67.6 65.2,66.03 v65.2,57.09
  Top 0.61: v65.13,28.51 65.13,35.52 67.36,37.75 67.36,52.86 66.6,53.62 v66.52,53.62
  Bottom 0.508: IC2.2 63.92,132.66 64.56,132.03 64.56,127.07 65.06,126.57 D1.A 63.66,126.57 v63.63,126.53 | D2.A 65.05,50.67 65.05,53.68 65.05,55.15 | 65.05,55.15 64.43,55.77 | 64.43,55.77 63.94,56.26 | 63.94,56.26 IC1.2 | 63.94,56.26 64.37,56.26 v65.2,57.09 65.05,56.94 65.05,56.31 | 65.05,56.31 65.05,55.15 | 65.05,56.31 64.51,55.77 64.43,55.77
  Bottom 0.61: D3.A 64.75,21.4 64.3,21.85 64.3,27.85 63.62,28.53 IC3.2 65.11,28.53 v65.13,28.51 | v66.52,53.62 65.11,53.62 65.05,53.68
GATE_HU  (via drill 0.35)  (1 unrouted)
  Top 0.508: R16.1 R17.1 R18.1 138.6,152.41 | R20.1 R21.1 97.96,139.83 R23.1
  Top 0.813: v73.57,124.28 96.18,124.28 97.96,126.06 97.96,139.83 | R23.1 R20.1 138.91,139.83 139.81,140.73 R19.1 138.6,152.41 R16.1
  Bottom 0.813: IC2.8 62.91,125.04 63.67,124.28 v73.57,124.28
GATE_HV  (via drill 0.35)
  Top 0.61: R1.1 206.79,152.41 R2.1 R3.1 240.68,152.45 R4.1 241.89,140.13 241.46,139.7 R5.1 R6.1 R47.1 185.17,139.7 R7.2 159.61,139.73 148.15,128.27 106.02,128.27 98.4,120.65 76.8,120.65 68.71,112.57 68.71,84.73 71.52,81.92 71.52,48.38 v72.28,47.62 72.32,47.66
  Bottom 0.61: IC1.8 62.94,48.64 63.96,47.62 v72.28,47.62
GATE_HW  (via drill 0.35)
  Top 0.61: R15.1 R13.1 R12.1 340.59,152.45 R11.1 341.94,140.69 340.9,139.65 340.2,139.65 R10.1 R9.1 R8.1 286.15,139.7 R14.2 278.84,139.5 271.63,132.29 271.63,42.08 256.2,26.65 77.4,26.65 v76.4,25.65
  Bottom 0.61: IC3.8 63.05,20.91 64.5,19.45 74.5,19.45 76.4,21.35 v76.4,25.65
GATE_LU  (via drill 0.35)
  Top 0.508: v64.69,133.93 71.46,133.93 72.06,133.33 72.06,122.07 v72.1,122.03
  Top 0.61: R56.2 83.34,40.2 R57.1 R55.1 R54.1 138.25,40.2 138.3,40.15 139.56,41.41 R53.1 138.66,52.65 126.45,52.65 R42.1 R41.1 R40.1 76.13,52.7 74.59,54.24 v74.59,66.55
  Bottom 0.508: v64.69,133.93 62.99,135.64 IC2.1
  Bottom 0.61: v72.1,122.03 73.1,121.03 73.1,78.03 74.59,76.54 v74.59,66.55
GATE_LV  (via drill 0.35)
  Top 0.61: R30.2 R31.1 R29.1 239.18,40.2 239.71,39.67 239.71,39.85 239.67,39.9 | 239.67,39.9 R28.1 | 239.67,39.9 241.01,39.9 242,40.88 R27.1 240.96,52.67 240.96,52.73 228.52,52.73 R26.1 R25.1 R24.1 161.3,52.7 149.03,64.97 79.5,64.97 76.21,68.26 v76.27,68.33 71.47,68.33 v71.43,68.28 | v66.57,66.62 66.57,58.71 v66.65,58.63
  Bottom 0.61: v71.43,68.28 68.23,68.28 v66.57,66.62 | v66.65,58.63 63.79,58.63 62.69,57.53 IC1.1
GATE_LW  (via drill 0.35)
  Top 0.61: R39.1 306.51,52.74 R37.1 328.05,52.7 R36.1 340.04,52.8 R35.1 341.14,40.99 340.35,40.2 R34.1 R33.1 317.35,39.7 317.3,39.65 316.75,40.2 R32.1 295.65,40.3 R38.2 278.85,40.3 260.7,22.15 74.4,22.15 73.3,23.25 73.3,30.55 71.9,31.95 v66.4,31.95
  Bottom 0.61: IC3.1 64.24,29.8 v66.4,31.95
GND  (via drill 0.35)  (4 unrouted)
  Top 0.406: 41.3,135.25 41.3,135.45 49.3,135.45 49.89,134.86 v49.89,132.57
  Top 0.61: C24.- C23.- 54.27,149.68 53.51,148.92 IPM2.2 | v49.89,132.57 49.89,124.2 v48.96,123.27 | v48.9,50.65 48.9,55.95 v49,56.05 | v48.5,30.45 v42.6,30.45
  Top 2.54: C17.- 43.35,147.25 42,147.25 42,136.65 40.9,136.65
  Bottom 0.61: IPM2.2 54.02,141.04 54.02,133.17 53.51,132.66 IC2.15 49.98,132.66 v49.89,132.57 | C17.- 44.28,136.69 C14.2 | 61.25,167.97 61.76,167.46 61.76,167.21 61.13,166.57 | 53.92,65.05 53.49,65.49 IPM1.2 53.92,66.28 | 53.92,65.05 53.92,56.77 53.41,56.26 IC1.15 49.21,56.26 v49,56.05 | C9.2 44.28,62.83 C11.- | C2.2 54.31,75.76 53.98,75.43 | 53.98,75.43 49.42,75.43 49.1,75.75 49.1,77.17 C1.2 48.96,77.37 v48.96,123.27 | 53.92,65.05 53.92,66.28 | 53.92,66.28 53.92,75.37 53.98,75.43 | C5.2 48.93,50.62 v48.9,50.65 | C21.- 44.28,32.99 C19.2 43.45,29.6 v42.6,30.45 | C29.2 330.24,185.57 R72.1 R73.1 R74.1 R71.1 | C6.2 53.13,42.26 IPM3.2 53.13,36.28 51.9,35.05 50.4,35.05 49.6,34.25 49.6,29.25 50.33,28.53 IC3.15 50.38,28.53 49.87,29.04 49.49,29.04 48.5,30.03 v48.5,30.45 | C12.2 49.46,14.99 49.8,14.65 55.1,14.65 54.79,14.96 C13.2
  Bottom 0.813: C22.2 54.33,164.98 55.92,166.57 61.13,166.57 62.06,166.57 IC4.3 | 62.78,166.7 67.6,166.7 68.49,165.81 68.49,150.95 67.22,149.68 C24.-
  pour Bottom (isolate 2.184): 438.92,177.6 434.84,181.68 140.07,181.68 140.07,184.98 143.12,188.03 443.88,188.03 454.86,177.06 454.86,22.01 441.96,9.12 419.97,9.12 426.85,16 426.85,36.07 432.19,41.4 439.29,41.4 447.17,49.28 447.17,168.67
  pour Bottom: 420.15,135.5 423.79,131.86 423.38,48.39 430.38,41.4 431.93,41.4 433.84,39.5 433.84,17.4 425.58,9.14 382.7,8.95 382.51,9.14 378.59,9.14 373.82,13.91 373.82,133.58 375.44,135.2 382.32,135.2 385.01,132.52 385.01,47.11 390.59,41.53 399.94,41.53 404.83,46.42 404.83,131.8 408.53,135.5
  pour Bottom: 374.91,19.25 371.71,16.05 72.9,16.05 68.45,11.6 71.2,8.85 384.1,8.85 377.5,15.45 377.5,18.35 376.6,19.25
  pour Bottom (isolate 3.81): 143.6,187.95 9.6,187.95 1.8,180.15 1.8,21.15 13.9,9.05 73.2,9.05 73.2,177.35 77.6,181.75 143.9,181.75 145.4,183.25 145.4,186.15
  pour Top (isolate 3.81): 9.7,187.85 76.9,187.85 78.1,186.65 77.2,10.15 76.4,9.35 14.3,9.35 1.8,21.85 1.8,179.95
N$1
  Bottom 0.61: IC1.12 48.6,52.45 47.16,51.01 R43.2
N$2
  Bottom 0.61: IC1.13 46.52,53.72 R44.2
N$3
  Top 0.61: Q1.1 185.3,154.37 R1.2
N$4
  Top 0.61: Q2.1 206.89,154.41 R2.2
N$5
  Top 0.61: Q3.1 228.48,154.38 R3.2
N$6
  Top 0.61: R4.2 249.4,151.24 Q4.1
N$7
  Top 0.61: R5.2 239.31,132.82 Q5.1
N$8  (1 unrouted)
  Top 0.61: R6.2 217.76,132.86
N$9
  Bottom 0.61: R59.2 46.8,22.95 48.56,24.72 IC3.12
N$10  (1 unrouted)
  Top 0.61: R8.2 296.95,132.2 297,132.15
N$11  (1 unrouted)
  Top 0.61: R9.2 318.45,132.83
N$12  (1 unrouted)
  Top 0.61: R10.2 340.15,132.86
N$13  (1 unrouted)
  Top 0.61: R11.2 350.14,151.1
N$14  (1 unrouted)
  Top 0.61: R12.2 329.25,158.79
N$15
  Top 0.61: 307.69,154.4 R13.2 307.65,158.8 Q12.1
N$16  (via drill 3 pad 6)
  other vias: 34.1,14.45
N$17
  Top 0.61: 286.11,154.41 R15.2 286.05,158.8 Q13.1
N$18  (via drill 3 pad 6)
  other vias: 34.2,94.85
N$19
  Bottom 0.61: IC1.14 46.89,54.99 R45.2
N$20
  Top 0.508: 83.22,156.66 R16.2
  Top 0.61: Q43.1 R16.2
N$21
  Top 0.61: R17.2 104.81,158.79 Q44.1
N$22
  Top 0.61: R18.2 126.4,158.94 Q14.1
N$23
  Top 0.61: R19.2 147.26,151.2 Q15.1
N$24
  Top 0.61: R20.2 137.2,132.79 Q16.1
N$25
  Top 0.61: R21.2 115.61,132.81 Q17.1
N$26
  Bottom 0.61: R48.1 62.44,43.52 C8.2
N$27
  Top 0.61: R23.2 94.02,132.83 Q18.1
N$28
  Bottom 0.61: R60.2 46.8,25.15 47.64,25.99 IC3.13
N$29
  Bottom 0.61: R61.2 46.21,27.26 IC3.14
N$30  (1 unrouted)
  Top 0.61: 185.26,59.27 R24.2
N$31
  Top 0.61: 206.89,54.64 R25.2 206.85,59.3 Q22.1
N$32
  Top 0.61: R26.2 228.49,59.26 Q23.1
N$33  (1 unrouted)
  Top 0.61: 249.38,51.63 R27.2
N$34  (1 unrouted)
  Top 0.61: 239.7,32.95 239.36,33.29 R28.2
N$35  (1 unrouted)
  Top 0.61: R29.2 217.71,33.3
N$36
  Bottom 0.61: C18.2 63.29,16.8 R63.1
N$37  (1 unrouted)
  Top 0.61: 196.11,33.29 R31.2
N$38  (via drill 3 pad 6)
  other vias: 7,94.85
N$39  (via drill 5 pad 9)
  other vias: 7.4,14.15
N$40
  Top 0.61: R32.2 295.75,33.3 Q28.1
N$41  (1 unrouted)
  Top 0.61: R33.2 317.35,33.28
N$42  (1 unrouted)
  Top 0.61: R34.2 338.95,33.29
N$43  (1 unrouted)
  Top 0.61: R35.2 349.08,51.7
N$44
  Top 0.61: Q32.1 328.1,54.75 R36.2
N$45
  Top 0.61: 307,54.15 R37.2 306.5,54.65 Q33.1
N$46  (via drill 5 pad 9)
  other vias: 7.2,183.75
N$47
  Top 0.61: R39.2 284.96,54.66 284.9,54.72 Q34.1
N$48
  Bottom 0.508: 410.6,135.2 410.72,135.07
N$49
  Bottom 0.508: 388.75,50.29 388.62,50.16
N$50  (1 unrouted)
  Top 0.61: 83.25,59.28 R40.2
N$51
  Top 0.61: R41.2 104.81,54.65 104.81,59.34 Q20.1
N$52
  Top 0.61: R42.2 Q35.1
N$53
  Top 0.61: R53.2 Q36.1
N$54
  Top 0.61: R54.2 137.2,38.24 137.09,38.24 136.8,37.95 137.2,37.55 Q38.1
N$55  (via drill 5 pad 9)
  other vias: 453,184.05
N$56  (via drill 5 pad 9)
  other vias: 452.4,14.15
N$57
  Top 3.1: 253,148.95 280.2,148.95
N$58
  Top 0.61: 196.09,137.79 R47.2 196.08,132.77 Q37.1
N$59
  Bottom 0.61: IC2.12 48.3,128.85 46.9,127.45 R49.2
N$60
  Bottom 0.61: IC2.13 46.74,130.12 R50.2
N$61
  Bottom 0.61: IC2.14 46.48,131.39 R51.2
N$63
  Top 0.61: Q39.1 R55.2
N$65
  Top 0.61: Q40.1 94,38.28 R57.2
N$67
  Bottom 0.508: C4.2 R58.1
SD  (via drill 0.35)
  Top 0.61: v40.18,128.69 40.2,128.67 v40.2,53.95 40.2,25.85 | 40.2,25.85 v40.4,25.65 | v9.4,39.25 9.4,28.35 11.9,25.85 40.2,25.85
  Bottom 0.61: R44.1 40.86,53.3 v40.2,53.95 | R50.1 44.08,130.06 41.35,130.06 40.18,128.89 v40.18,128.69 | R60.1 40.9,25.15 v40.4,25.65 | J1.9 8.55,45 9.4,44.15 v9.4,39.25
U  (via drill 0.6, 10.5 pad 17)
  Top 0.61: 80.45,130.12 83.08,132.75 Q18.3 83.08,136.58 83.12,136.62
  Top 0.813: v73.7,130.12 80.45,130.12
  Top 1.016: R22.1 84.66,138.16 83.12,136.62
  Bottom 0.813: v73.7,130.12 69.95,130.12 R52.2
  other vias: 159.92,99.38
  pour Bottom: 135.42,157.05 139.87,157.05 140.38,157.55 140.38,163.9 139.11,165.17 78.14,165.17 75.48,162.51 75.48,130.38 79.03,126.82 169.17,126.82 170.82,128.47 170.82,140.41 170.57,140.66 146.21,140.66 145.75,140.2 145.75,137.45 147.13,136.07 148.63,136.07 148.63,132.79 145.2,129.36 130.47,129.36 128.18,131.65 128.18,134.06 126.91,135.33 124.63,135.33 123.99,134.69 123.99,130.38 122.59,128.98 107.74,128.98 106.59,130.12 106.59,133.8 105.07,135.33 102.91,135.33 101.77,134.19 101.77,130.38 100.37,128.98 87.03,128.98 84.88,131.14 84.88,133.8 83.35,135.33 80.05,135.33 79.41,135.96 79.41,161.36 80.69,162.63 90.84,162.63 92.37,161.11 92.37,157.93 93.38,156.92 97.19,156.92 97.83,157.55 97.83,162 98.47,162.63 112.44,162.63 113.96,161.11 113.96,157.93 114.98,156.92 118.79,156.92 119.42,157.55 119.42,162 120.05,162.63 133.39,162.63 135.42,160.6
  pour Bottom: 152.06,47.75 152.06,45.47 151.04,44.45 143.17,44.45 141.77,43.05 141.77,37.08 141.01,36.32 135.3,36.32 134.53,35.56 134.53,32.13 133.77,31.37 131.1,31.37 129.96,32.51 129.96,35.18 128.82,36.32 113.96,36.32 112.82,35.18 112.82,32.13 112.05,31.37 109.39,31.37 108.24,32.51 108.24,35.18 107.1,36.32 91.86,36.32 91.1,35.56 91.1,32.51 89.96,31.37 87.67,31.37 86.53,32.51 86.53,35.18 83.48,38.23 83.48,55.75 84.24,56.51 85.38,56.51 86.15,57.28 86.15,60.32 86.91,61.09 89.58,61.09 90.34,60.32 90.34,57.28 91.1,56.51 107.1,56.51 107.86,57.28 107.86,60.32 108.62,61.09 111.29,61.09 112.05,60.32 112.05,57.28 112.82,56.51 128.82,56.51 129.2,56.9 129.2,59.94 130.34,61.09 132.63,61.09 133.77,59.94 133.77,56.9 134.53,56.13 141.39,56.13 142.53,54.99 142.53,49.28 143.3,48.51 151.3,48.51
  pour Bottom: 168.32,44.45 170.7,46.82 170.7,129.11 168.66,131.14 147.87,131.14 144.82,128.09 82.84,128.09 79.41,131.52 76.24,131.52 75.48,130.76 75.48,72.14 78.91,68.71 140.63,68.71 144.06,65.28 144.06,58.04 145.96,56.13 149.39,56.13 150.15,55.37 150.15,48.89 149.39,48.13 144.82,48.13 144.82,46.61 146.98,44.45
U_HIN  (via drill 0.35)
  Top 0.61: v13,61.25 13,122.75 17.6,127.35 23.9,127.35 v24,127.45
  Bottom 0.61: J1.3 12.19,60.24 13,61.05 v13,61.25 | R49.1 v24,127.45
U_LIN  (via drill 0.35)
  Top 0.61: v16.9,60.95 16.9,119.85 v20.4,123.35
  Bottom 0.61: J1.4 13.65,57.7 v16.9,60.95 | v20.4,123.35 20.4,129.65 22.39,131.65 R51.1
V  (via drill 0.35, 10.5 pad 17)
  Top 0.61: Q37.3 185.2,137.97 R7.1 161.1,138.03 149.36,126.29 107.01,126.29 98.37,117.65 81.8,117.65 73.27,109.12 v73.27,75.19
  Bottom 0.61: R46.2 71.89,53.21 73.27,54.59 v73.27,75.19
  other vias: 259.78,99.38
  pour Bottom (isolate 2.184): 237.5,160.86 237.5,157.81 238.39,156.92 242.2,156.92 243.47,158.19 243.47,163.14 241.31,165.3 180.77,165.3 177.81,162.34 177.81,125.93 177.93,125.8 253.12,125.8 254.01,126.69 254.01,141.07 247.66,141.07 247.66,138.12 248.55,137.23 248.55,130.76 246.9,129.11 231.78,129.11 230.39,130.5 230.39,133.3 229.12,134.57 226.7,134.57 225.69,133.55 225.69,130.63 224.16,129.11 209.3,129.11 208.67,129.74 208.67,134.06 208.03,134.69 204.6,134.69 203.08,133.17 203.08,129.49 202.7,129.11 188.09,129.11 187.59,129.61 187.59,129.74 187.21,130.12 187.21,133.55 186.06,134.69 181.24,134.69 180.47,135.46 180.47,159.59 182.76,161.87 192.79,161.87 194.32,160.35 194.32,157.93 195.33,156.92 199.27,156.92 200.29,157.93 200.29,161.24 201.68,162.63 214,162.63 215.91,160.73 215.91,157.93 216.92,156.92 217.05,157.05 220.35,157.05 222.13,158.82 222.13,160.86 223.91,162.63 235.72,162.63
  pour Bottom: 254.64,47.75 254.64,45.21 253.88,44.45 246.77,44.45 244.99,42.67 244.99,37.59 243.97,36.58 237.62,36.58 236.61,35.56 236.61,31.75 236.35,31.5 232.8,31.5 232.04,32.26 232.04,35.56 231.02,36.58 215.53,36.58 214.76,35.81 214.76,32.26 214,31.5 211.21,31.5 210.45,32.26 210.45,35.81 209.94,36.32 194.19,36.32 193.3,35.43 193.3,32.13 192.54,31.37 189.87,31.37 188.73,32.51 188.73,35.56 187.97,36.32 184.16,36.32 183.4,37.08 183.4,55.75 184.16,56.51 186.82,56.51 187.97,57.66 187.97,60.32 188.73,61.09 191.78,61.09 192.54,60.32 192.54,57.28 194.06,55.75 208.92,55.75 209.68,56.51 209.68,60.32 210.45,61.09 213.11,61.09 214.26,59.94 214.26,56.51 215.02,55.75 230.64,55.75 231.4,56.51 231.4,59.94 232.54,61.09 234.83,61.09 235.97,59.94 235.97,56.51 236.74,55.75 245.12,55.75 245.88,54.99 245.88,48.89 246.26,48.51 253.88,48.51
  pour Bottom (isolate 2.184): 248.97,141.16 271.33,141.16 272.46,140.03 272.46,44.9 272.01,44.45 246.77,44.45 245.62,45.59 245.62,47.75 246.13,48.26 254.26,48.26 254.82,48.81 254.82,67.44 249.26,72.99 177.61,72.99 177.61,126.75 179.58,128.72 246.9,128.72 249.18,131.01 249.18,137.23 247.53,138.88 247.53,139.72
V_LIN
  Bottom 0.61: J1.6 36.67,52.62 39.72,55.68 R45.1
VBU
  Bottom 0.508: C15.1 69.85,133.25 C3.1 69.85,140.07 68.37,141.55 IPM2.6 63.79,141.68 63.79,142.31 63.03,143.08 57.19,143.08 56.94,142.82 56.94,127.58 58.21,126.31 IC2.7
VBV
  Bottom 0.508: IC1.7 58.29,49.91 56.55,51.65 56.55,66.4 57.55,67.4 62.55,67.4 63.29,66.67 IPM1.6 63.37,65.4 69.3,65.4 70.44,64.26 C7.1 70.44,56.35 C10.1
VBW
  Bottom 0.61: C20.1 70.44,27.74 C16.1 70.44,34.71 67.83,37.32 IPM3.6 63.29,37.67 62,38.95 57.1,38.95 56.6,38.45 56.6,23.55 58,22.15 61.26,22.15 IC3.7
VCC  (via drill 0.35)
  Top 0.508: v58.3,48.65 58.3,54.15 v59.05,54.9 59.14,54.99 59.14,63.66 59.91,64.43 v59.91,68.12
  Top 0.61: v58.3,124.65 58.3,130.65 v59.05,131.4 | v59.4,40.05 60,39.45 60,35.85 58.7,34.55 58.7,27.65 | v58.7,20.85 58.7,26.85 | 58.7,26.85 58.7,27.65 | 58.7,27.65 v59.1,27.25 58.7,26.85
  Bottom 0.508: C8.1 58.35,48.6 v58.3,48.65 | v59.05,54.9 59.14,54.99 IC1.3 | C4.1 58.31,69.72 v59.91,68.12
  Bottom 0.61: v58.3,124.65 58.3,101.67 58.31,101.66 C4.1 | v59.05,131.4 IC2.3 | C18.1 58.7,17.21 v58.7,20.85 | v59.1,27.25 IC3.3 | C8.1 58.35,41.1 v59.4,40.05
VSCOM  (via drill 0.35)  (1 unrouted)
  Top 0.61: v61.7,68.67 61.79,68.58 61.79,60.73 63.42,59.1 v63.42,45.92 63.24,45.92 61.59,44.27 61.59,20.25 63.5,18.34 v64.79,18.34 | v73.96,43.11 74.55,43.11 79.26,38.4 R56.1 83.1,38.26 Q40.3 | 185.2,38.44 R30.1 185.26,33.31 Q27.3 | R38.1 284.8,33.33
  Bottom 0.61: R58.2 64.74,71.46 61.95,68.67 v61.7,68.67 | v63.42,45.92 64.35,44.99 R48.2 64.81,43.07 73.92,43.07 v73.96,43.11 | R63.2 65.21,17.92 v64.79,18.34
  Bottom 1.27: 176.64,40.79 178.82,38.61
  pour Bottom: 136.56,57.4 139.74,57.4 140.38,58.04 140.38,63.12 138.47,65.02 77.38,65.02 75.35,62.99 75.35,29.72 77.51,27.56 149.27,27.56 151.81,30.1 151.81,41.53 150.54,42.8 146.09,42.8 144.82,41.53 144.82,32 142.92,30.1 128.95,30.1 127.67,31.37 127.67,33.27 126.4,34.54 123.23,34.54 122.59,33.91 122.59,30.73 121.96,30.1 107.36,30.1 106.72,30.73 106.72,33.91 105.45,35.18 101.64,35.18 101,34.54 101,30.73 100.37,30.1 85.77,30.1 85.13,30.73 85.13,33.91 81.95,37.08 80.05,37.08 80.05,60.58 81.95,62.48 90.84,62.48 92.11,61.21 92.11,58.67 93.38,57.4 97.83,57.4 98.47,58.04 98.47,61.21 99.73,62.48 113.07,62.48 113.7,61.85 113.7,58.67 114.98,57.4 118.79,57.4 120.05,58.67 120.05,61.21 120.69,61.85 134.66,61.85 135.3,61.21 135.3,58.67
  pour Bottom: 238.64,57.4 242.45,57.4 243.09,58.04 243.09,63.75 241.81,65.02 177.68,65.02 176.41,63.75 176.41,29.46 178.95,26.92 251.98,26.92 254.51,29.46 254.51,41.53 253.25,42.8 248.8,42.8 247.53,41.53 247.53,31.37 246.26,30.1 231.02,30.1 230.39,30.73 230.39,33.91 229.12,35.18 225.31,35.18 224.67,34.54 224.67,30.73 224.04,30.1 209.43,30.1 208.8,30.73 208.8,33.91 207.53,35.18 203.08,35.18 202.45,34.54 202.45,30.73 201.81,30.1 188.48,30.1 187.21,31.37 187.21,33.91 185.94,35.18 180.22,35.18 179.59,35.81 179.59,62.48 180.22,63.12 193.56,63.12 194.19,62.48 194.19,58.67 195.46,57.4 199.27,57.4 200.54,58.67 200.54,62.48 201.18,63.12 215.15,63.12 215.78,62.48 215.78,58.67 217.05,57.4 220.86,57.4 222.13,58.67 222.13,62.48 222.77,63.12 236.1,63.12 237.37,61.85 237.37,58.67
  pour Bottom: 338.18,57.4 341.99,57.4 342.62,58.04 342.62,63.75 341.35,65.02 279.12,65.02 277.85,63.75 277.85,28.83 279.75,26.92 350.88,26.92 354.05,30.1 354.05,41.53 352.78,42.8 348.59,42.8 347.06,41.27 347.06,31.37 345.16,29.46 331.19,29.46 329.92,30.73 329.92,33.91 328.65,35.18 324.84,35.18 323.57,33.91 323.57,30.73 322.3,29.46 309.6,29.46 308.33,30.73 308.33,33.91 307.06,35.18 303.25,35.18 301.98,33.91 301.98,30.1 301.35,29.46 288.01,29.46 286.74,30.73 286.74,33.91 285.47,35.18 282.3,35.18 281.03,36.45 281.03,61.85 282.3,63.12 293.09,63.12 293.73,62.48 293.73,58.67 295,57.4 298.81,57.4 300.07,58.67 300.07,61.85 301.35,63.12 314.68,63.12 315.31,62.48 315.31,58.67 316.59,57.4 320.4,57.4 321.67,58.67 321.67,61.85 322.94,63.12 336.27,63.12 336.91,62.48 336.91,58.67
  pour Bottom: 354.2,19.15 353.7,18.65 81.8,18.65 79.3,21.15 79.3,27.65 79.8,28.15 143.3,28.15 150.3,35.15 150.3,42.65 150.6,42.95 176,42.95 179.5,39.45 179.5,28.65 184.9,28.65 185.2,28.95 250,28.95 251,29.95 251,39.55 253.3,41.85 253.3,42.85 253.4,42.95 279.1,42.95 279.3,43.15 279.3,32.35 282.2,29.45 347.7,29.05 353.1,29.05 354.2,30.15
VSU
  Bottom 0.508: IPM2.4 58.59,140.79 | 58.59,140.79 58.59,140.41 | 59.86,139.14 60.24,139.14 | 60.24,139.14 67.22,139.14 68.15,138.21 C3.2 66.84,134.52 C15.2 66.84,130.51 67.35,129.99 R52.1 68.11,129.81 68.11,127.58 69.76,125.93 69.78,125.95 D1.K | 58.59,140.41 58.91,140.09 | 58.91,140.09 58.97,140.03 | 58.97,140.03 59.6,139.39 | 59.6,139.39 59.86,139.14 | IC2.6 58.84,127.58 57.95,128.47 57.95,139.14 | 57.95,139.14 57.95,139.39 | 57.95,139.39 57.95,139.77 | 57.95,139.77 58.14,139.96 | 58.14,139.96 58.59,140.41 | 57.95,139.14 58.21,139.14 | 58.21,139.14 59.86,139.14 | 59.6,139.39 58.71,139.39 | 58.71,139.39 58.4,139.71 | 58.4,139.71 58.14,139.96 | 58.91,140.09 58.91,139.58 58.71,139.39 | 58.97,140.03 58.65,139.71 58.4,139.71 | 57.95,139.77 57.95,140.92 | 57.95,140.92 IPM2.4 | 58.59,140.41 58.46,140.41 58.27,140.6 | 58.27,140.6 57.95,140.92 | IPM2.4 58.27,141.23 58.27,140.6 | 58.59,140.79 60.24,139.14 | 58.21,139.14 57.95,139.39
VSV
  Bottom 0.508: IPM1.4 58.21,64.34 | 58.21,64.34 58.21,63.74 | 58.21,63.74 58.21,63.18 | 58.21,63.18 58.21,51.75 58.8,51.15 61.25,51.15 IC1.6 | 68.74,58.4 C7.2 68.74,62.9 67.9,63.74 58.83,63.74 | 68.74,58.4 68.74,56.59 | 68.74,56.59 68.05,55.9 67.61,55.9 C10.2 | 68.43,53.4 R46.1 68.43,50.54 68.3,50.4 68.67,50.04 D2.K | 68.43,53.4 68.43,58.1 68.74,58.4 | 68.74,56.59 68.74,53.71 68.43,53.4 | 58.83,63.74 58.23,64.34 58.21,64.34 | 58.21,63.74 58.83,63.74 | 58.83,63.74 58.27,63.18 58.21,63.18
VSW
  Bottom 0.61: IPM3.4 58.21,35.95 | 58.21,35.95 58.21,35.15 | 58.21,35.15 58.21,34.36 | 58.21,34.36 58.21,24.55 59.3,23.45 IC3.6 | 67.93,24.72 67.4,24.72 67.4,25.25 | 67.93,24.72 R62.1 68.43,22.02 69.05,21.4 D3.K | 67.4,25.25 C20.2 67.4,29.55 67.95,30.1 C16.2 68.74,33.41 67,35.15 59,35.15 | 67.4,25.25 67.93,24.72 | 58.21,35.15 59,35.15 | 59,35.15 58.21,34.36 | 59,35.15 58.21,35.95
W  (via drill 0.35, 10.5 pad 17)
  Top 0.61: v74.4,24.65 257.9,24.65 275.05,41.8 275.05,131.08 281.72,137.75 286,137.75 R14.1 285.95,132.3 286.1,132.15 286.1,132.75 Q7.3
  Bottom 0.61: R62.2 74.33,24.72 v74.4,24.65
  other vias: 354.8,99.38
  pour Bottom: 338.32,157.91 339.19,157.05 342.37,157.05 343,157.68 343,163.14 341.99,164.16 279.5,164.16 278.1,162.76 278.1,126.95 279.5,125.55 352.53,125.55 354.18,127.2 354.18,140.28 353.9,140.56 348.68,140.56 348.08,139.96 348.08,130.25 346.3,128.47 332.71,128.47 331.19,129.99 331.19,133.68 330.3,134.57 327.25,134.57 325.98,133.3 325.98,129.99 325.35,129.36 309.6,129.36 309.35,129.61 309.35,133.55 308.2,134.69 305.41,134.69 304.39,133.68 304.39,130.12 303.88,129.61 288.39,129.61 287.76,130.25 287.76,133.68 286.74,134.69 283.31,134.69 282.68,135.33 282.68,160.35 284.2,161.87 294.11,161.87 295.25,160.73 295.25,157.93 296.26,156.92 300.33,156.92 300.96,157.55 300.96,160.98 301.73,161.74 316.33,161.74 316.71,161.36 316.71,158.06 317.86,156.92 322.3,156.92 322.81,157.43 322.81,160.6 323.82,161.62 337.92,161.62 338.47,161.07
  pour Bottom: 354.18,47.75 354.18,45.08 353.42,44.32 345.03,44.32 343.89,43.18 343.89,37.08 342.75,35.94 337.41,35.94 336.27,34.8 336.27,32.13 335.51,31.37 332.84,31.37 331.32,32.89 331.32,35.94 330.56,36.7 315.31,36.7 314.55,35.94 314.55,32.13 313.79,31.37 311.12,31.37 309.98,32.51 309.98,35.94 309.22,36.7 294.36,36.7 293.22,35.56 293.22,32.13 292.45,31.37 289.41,31.37 288.65,32.13 288.65,35.18 287.12,36.7 284.07,36.7 283.69,37.08 283.69,55.75 284.45,56.51 286.36,56.51 287.5,57.66 287.5,60.32 288.26,61.09 291.31,61.09 292.07,60.32 292.07,56.9 292.84,56.13 308.46,56.13 309.22,56.9 309.22,59.94 310.36,61.09 312.65,61.09 313.79,59.94 313.79,56.9 314.55,56.13 330.17,56.13 330.94,56.9 330.94,60.32 331.7,61.09 334.37,61.09 335.51,59.94 335.51,56.9 336.27,56.13 342.37,56.13 344.4,54.1 344.4,49.53 345.41,48.51 353.42,48.51
  pour Bottom: 349.08,44.29 362.25,44.29 365,47.03 365,133.86 355.06,141.04 348.08,141.04 348.08,129.99 345.03,126.95 278.77,126.95 278.77,71.56 349.54,71.56 357.84,63.26 357.84,50.49 355.83,48.48 347.59,48.48 347.44,48.34 347.44,45.92
W_HIN  (via drill 0.35)
  Top 0.61: v13.3,39.15 13.3,30.65 15,28.95 v33.7,28.95
  Bottom 0.61: J1.7 9.97,50.08 13.3,46.75 v13.3,39.15 | v33.7,28.95 33.7,25.75 36.5,22.95 R59.1
W_LIN  (via drill 0.35)
  Top 0.61: v36.6,27.35 13.6,27.35 11.5,29.45 v11.5,39.25
  Bottom 0.61: J1.8 9.51,47.54 11.5,45.55 v11.5,39.25 | v36.6,27.35 44.42,27.35 R61.1

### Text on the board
tValues: W
Descript: + | U | V | -

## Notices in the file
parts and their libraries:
con-headers-jp: Copyright (C) 2008, Bob Starr
